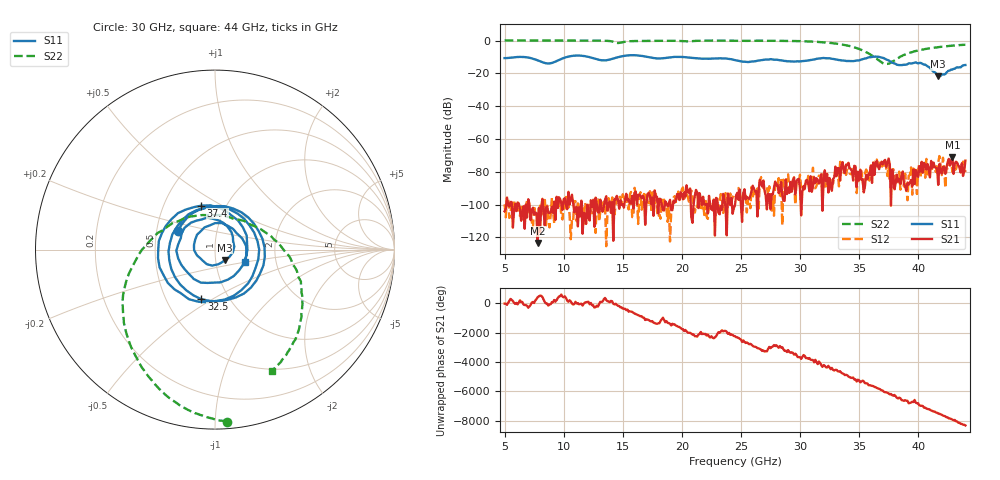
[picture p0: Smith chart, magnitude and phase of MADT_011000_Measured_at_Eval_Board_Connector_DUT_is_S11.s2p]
!MADT-011000 Measured on a PCB AND NOT DE-EMBEDDED
!S11 is the device on the evaluation board.  Reference plane is the connector.
!Data should be considered typical for reference purposes
!Keysight Technologies,N5247A,US50470148,A.10.40.12
!Date: Friday, October 07, 2016 08:54:41
!Correction: S11(Full 2 Port(1,2))
!S21(Full 2 Port(1,2))
!S12(Full 2 Port(1,2))
!S22(Full 2 Port(1,2))
!S2P File: Measurements: S11, S21, S12, S22:
# Hz S  RI  R 50
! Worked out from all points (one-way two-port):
!   391 points, 5 GHz to 44 GHz, reference 50 ohm
!   highest |S21| = -71.07 dB at 42.9 GHz (marker M1); lowest = -123.5 dB at 7.8 GHz (marker M2)
!   lowest |S11| = -21.9 dB at 41.7 GHz (marker M3), VSWR 1.17, Z = 55.5 - j6.46 ohm
!   |S11| at or under -10 dB: start of sweep to 10.3 GHz; 19.97 GHz to 36.1 GHz (16.13 GHz wide, 57.5 % of centre); 36.7 GHz to end of sweep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
!   |S22| runs from -14.3 to 0.0 dB; largest |S21 - S12| = 0.00022
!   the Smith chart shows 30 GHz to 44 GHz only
!   S11 on the Smith chart (normalised r, x): 30 GHz: 0.64, +0.14; 32.5 GHz: 0.74, -0.45; 37.4 GHz: 0.77, +0.40; 44 GHz: 1.38, -0.20
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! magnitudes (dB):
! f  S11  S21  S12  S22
! 5 GHz  -10.7  -104.1  -99.9  0.0
! 7.8 GHz  -12.1  -123.5  -118.5  0.0
! 11.5 GHz  -9.3  -97.7  -103.5  0.0
! 18 GHz  -10.9  -105.5  -107.7  -0.2
! 24.5 GHz  -11.9  -100.4  -93.9  -0.2
! 30 GHz  -12.7  -90.5  -81.8  -0.3
! 31 GHz  -11.8  -92.3  -85.6  -0.7
! 32.5 GHz  -10.8  -83.8  -85.6  -1.4
! 36.3 GHz  -9.9  -81.9  -73.9  -10.1
! 36.5 GHz  -9.9  -73.4  -72.6  -11.1
! 37.4 GHz  -11.8  -74.5  -82.7  -14.2
! 37.5 GHz  -12.1  -72.0  -75.3  -14.1
! 37.7 GHz  -13.1  -100.7  -79.1  -13.4
! 40.6 GHz  -14.7  -76.2  -83.7  -5.2
! 40.7 GHz  -15.3  -78.7  -72.2  -5.1
! 41.1 GHz  -17.5  -73.4  -79.5  -4.6
! 41.7 GHz  -21.9  -88.1  -74.4  -4.0
! 42.3 GHz  -20.4  -81.3  -90.0  -3.5
! 42.8 GHz  -17.7  -73.4  -73.2  -3.2
! 42.9 GHz  -17.8  -71.1  -80.2  -3.1
! 43 GHz  -17.3  -81.3  -77.0  -3.1
! 44 GHz  -14.9  -73.2  -80.2  -2.6
